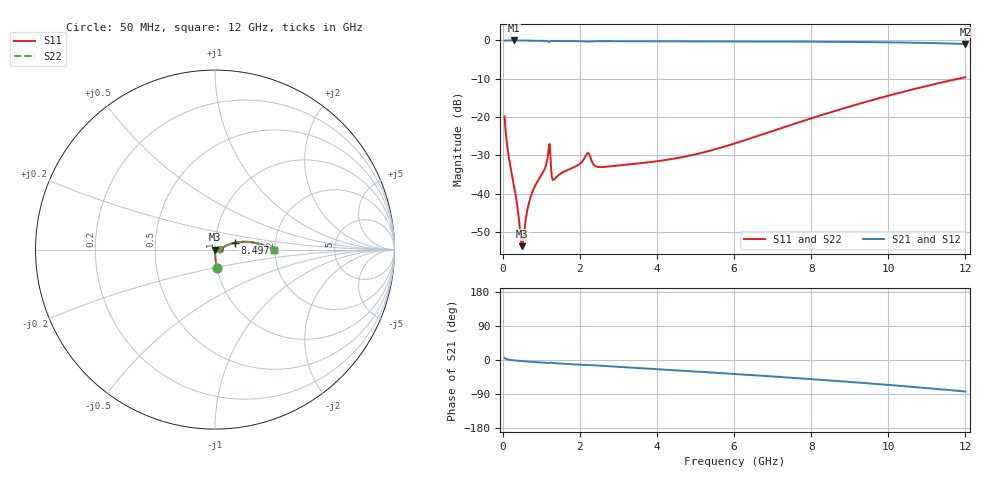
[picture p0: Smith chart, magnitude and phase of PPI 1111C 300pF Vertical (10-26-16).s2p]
# GHz S MA R 50
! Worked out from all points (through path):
!   1601 points, 50 MHz to 12 GHz, reference 50 ohm
!   highest |S21| = 0.00 dB at 281.5 MHz (marker M1); lowest = -0.9 dB at 12 GHz (marker M2)
!   group delay of S21, straight-line fit = 18.8 ps
!   lowest |S11| = -53.7 dB at 505.6 MHz (marker M3), VSWR 1.00, Z = 50.2 - j0.0621 ohm
!   |S11| at or under -10 dB: start of sweep to 11.82 GHz
!   |S22| runs from -53.7 to -9.6 dB; largest |S21 - S12| = 0
!   S11 on the Smith chart (normalised r, x): 50 MHz: 1.00, -0.20; 8.497 GHz: 1.24, +0.10; 12 GHz: 1.99, -0.02
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0.05  0.1013 -84.2  0.9943 5.5  0.9943 5.5  0.1013 -84.2
0.1620312  0.02934 -88.3  0.9991 0.7  0.9991 0.7  0.02934 -88.3
0.2815313  0.01372 -89.0  0.9994 -0.9  0.9994 -0.9  0.01372 -89.0
0.4607812  0.002928 -62.9  0.9985 -2.6  0.9985 -2.6  0.002928 -62.9
0.5055937  0.002066 -17.4  0.998 -3.0  0.998 -3.0  0.002066 -17.4
0.5429375  0.002746 18.5  0.9974 -3.3  0.9974 -3.3  0.002746 18.5
0.6400313  0.006156 41.5  0.9956 -4.1  0.9956 -4.1  0.006156 41.5
0.7221875  0.00899 42.9  0.9939 -4.7  0.9939 -4.7  0.00899 42.9
1.080688  0.02056 34.6  0.9845 -7.3  0.9845 -7.3  0.02056 34.6
1.177781  0.03252 27.8  0.9734 -8.2  0.9734 -8.2  0.03252 27.8
1.222594  0.04232 -13.7  0.9579 -7.1  0.9579 -7.1  0.04232 -13.7
1.297281  0.01526 -10.6  0.9847 -7.7  0.9847 -7.7  0.01526 -10.6
1.334625  0.01534 0.5  0.9847 -8.1  0.9847 -8.1  0.01534 0.5
2.044156  0.02572 8.9  0.9759 -12.8  0.9759 -12.8  0.02572 8.9
2.201  0.03377 -4.2  0.9665 -13.5  0.9665 -13.5  0.03377 -4.2
2.49975  0.02226 -12.6  0.9776 -15.0  0.9776 -15.0  0.02226 -12.6
4.038312  0.02668 -3.0  0.9749 -24.4  0.9749 -24.4  0.02668 -3.0
6.025  0.0454 14.9  0.971 -37.0  0.971 -37.0  0.0454 14.9
8.019156  0.09681 20.1  0.9634 -50.6  0.9634 -50.6  0.09681 20.1
8.497156  0.1152 19.2  0.9603 -54.1  0.9603 -54.1  0.1152 19.2
10.01331  0.1907 12.9  0.9447 -65.8  0.9447 -65.8  0.1907 12.9
12  0.3309 -0.6  0.901 -83.1  0.901 -83.1  0.3309 -0.6
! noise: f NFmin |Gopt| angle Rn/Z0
0.05  0.0005204  0.9024  0.3313  0.001167
1.372  0.01418  0.9021  8.224  0.03155
2.701  0.02378  0.8874  16.1  0.04502
4.031  0.03035  0.8721  23.79  0.04899
5.36  0.03599  0.8614  31.25  0.05163
6.682  0.04125  0.8548  38.39  0.05414
8.012  0.04648  0.8517  45.24  0.05699
9.341  0.05183  0.8516  51.75  0.06038
10.67  0.05749  0.8541  57.91  0.06452
12  0.06361  0.8586  63.71  0.06962
